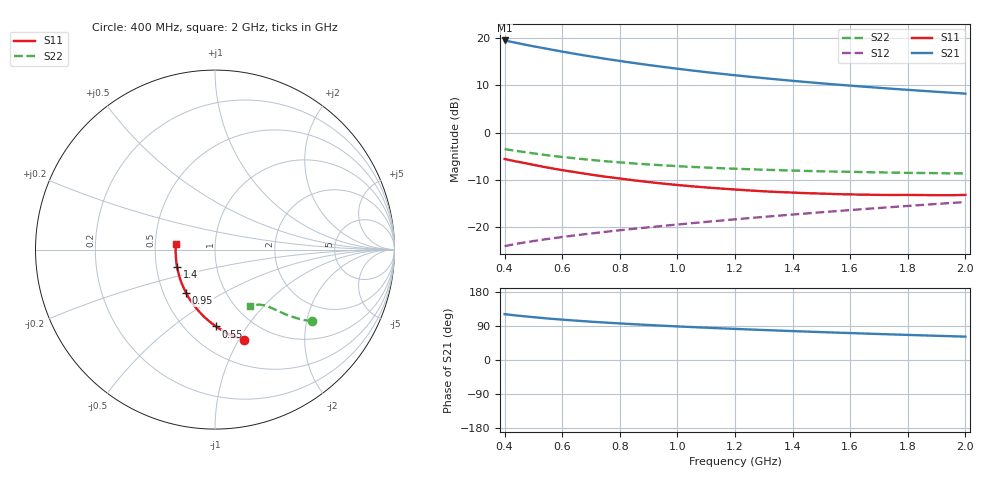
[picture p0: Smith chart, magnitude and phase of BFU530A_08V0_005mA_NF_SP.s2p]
! Filename:  P:\Prog\Test\Noise\ATS_data\Testdata_Net\06 Compressed Noise after Statistics\BFU530A_APG2013_33_A05_08p0V_005mA_NF_CM01_D.sf
! Date/Time: Tue 16/Apr/2013 15:10:58
! BFU530A_APG2013_33_A05_08p0V_1to25mA_NF_CM01_Bias4_R.sf
! Noise Parameter Data File
! BFU530A_APG2013_33_A05_08p0V_1to25mA_NF_CM01
! Date/time: Fri Apr 12 16:45:05 2013
! VAR V_out= 8.001000
! VAR I_out= 4.995000
! VAR V_in= 0.813500
! VAR I_in= 0.051000
! Device data file deembeded for feedlines and parallel
! Original file: \06 Compressed Noise after Statistics\BFU530A_APG2013_33_A05_08p0V_005mA_NF_CM01_R.sf
! Feed-files: PR017V01_150413_Feed1.s2p, PR017V01_150413_Feed2.s2p
! Parallel-file: PR017V01_150413_Par.s2p
# MHz S MA R 50
!  Freq-MHz  S11-mag  S11-arg  S21-mag  S21-arg  S12-mag  S12-arg  S22-mag  S22-arg
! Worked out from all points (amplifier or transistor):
!   37 points, 400 MHz to 2 GHz, reference 50 ohm
!   highest |S21| = 19.5 dB at 400 MHz (marker M1)
!   |S21| within 3 dB of that: start of sweep to 661.1 MHz
!   unconditionally stable (mu >= 1): 1.639 GHz to end of sweep
!   at 500 MHz: K = 0.60, MSG = 20.6 dB, |S12| = -22.9 dB
!   at 1.1 GHz: K = 0.91, MSG = 15.8 dB, |S12| = -18.8 dB
!   at 2 GHz: K = 1.01, MAG = 10.8 dB, |S12| = -14.7 dB
!   lowest NFmin = 0.60 dB at 420 MHz
!   S11 on the Smith chart (normalised r, x): 400 MHz: 0.76, -1.05; 550 MHz: 0.70, -0.73; 950 MHz: 0.65, -0.34; 1.4 GHz: 0.64, -0.13; 2 GHz: 0.64, +0.04
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400  0.5272 -72.2  9.467 121.0  0.06321 60.5  0.6722 -36.3
420  0.5123 -74.7  9.195 119.2  0.06507 60.1  0.6575 -37.1
440  0.4975 -77.2  8.939 117.5  0.06679 59.7  0.6439 -37.8
480  0.4715 -81.7  8.441 114.5  0.07003 59.1  0.618 -39.0
500  0.4581 -83.9  8.214 113.0  0.07164 58.9  0.6063 -39.5
550  0.428 -89.3  7.703 109.5  0.07531 58.5  0.5776 -40.7
600  0.4029 -94.1  7.219 106.5  0.07902 58.3  0.5545 -41.6
650  0.3811 -98.8  6.789 103.8  0.08266 58.2  0.5346 -42.5
700  0.3609 -103.3  6.407 101.1  0.08609 58.2  0.5164 -43.2
750  0.3433 -107.6  6.057 98.8  0.08961 58.3  0.5002 -43.8
800  0.3285 -111.8  5.748 96.5  0.09312 58.5  0.4866 -44.4
850  0.3138 -115.9  5.465 94.4  0.09657 58.6  0.4735 -44.9
900  0.3014 -119.9  5.207 92.4  0.1001 58.8  0.4626 -45.4
950  0.2901 -123.7  4.973 90.5  0.1035 59.1  0.4527 -46.0
1050  0.2717 -131.0  4.559 86.9  0.1106 59.6  0.4355 -46.8
1200  0.2511 -141.6  4.058 82.1  0.1216 60.2  0.4167 -48.3
1300  0.2405 -148.3  3.783 79.1  0.129 60.5  0.407 -49.4
1400  0.233 -154.8  3.543 76.3  0.1366 60.8  0.3984 -50.5
1500  0.2274 -161.2  3.334 73.6  0.1443 61.0  0.3914 -51.6
1650  0.2215 -169.8  3.068 69.8  0.1562 61.2  0.3837 -53.6
1750  0.22 -175.4  2.914 67.4  0.1643 61.3  0.379 -54.8
2000  0.2202 172.0  2.596 61.6  0.1851 61.1  0.3714 -58.6
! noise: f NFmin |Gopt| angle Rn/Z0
400  0.6308  0.2002  23.41  0.1252
460  0.603  0.1728  34.99  0.1115
600  0.7108  0.1928  33.51  0.1252
800  0.6866  0.1753  59.82  0.103
1000  0.718  0.1781  77.35  0.0954
1200  0.7608  0.1785  92.36  0.0927
1400  0.807  0.1835  109.5  0.083
1600  0.7747  0.1794  130.6  0.0803
1800  0.8017  0.2079  147.9  0.066
2000  0.7929  0.2241  165.3  0.0639
